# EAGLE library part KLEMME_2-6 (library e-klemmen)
Klemme 2 6
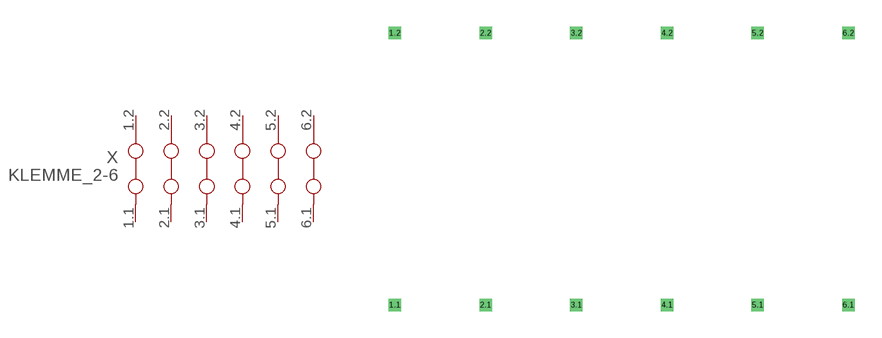
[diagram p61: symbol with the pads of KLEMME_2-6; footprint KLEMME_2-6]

Designator prefix X

## KLEMME_2-6  [KLEMME_2-6]
1.1  1.1  pas
1.2  1.2  pas
2.1  2.1  pas
2.2  2.2  pas
3.1  3.1  pas
3.2  3.2  pas
4.1  4.1  pas
4.2  4.2  pas
5.1  5.1  pas
5.2  5.2  pas
6.1  6.1  pas
6.2  6.2  pas

## Footprint KLEMME_2-6 (pad centres in mm)
Dummy
drill 0.2 pad 0.6 square: 1.1 0,-7.62; 1.2 0,7.62; 2.1 5.08,-7.62; 2.2 5.08,7.62; 3.1 10.16,-7.62; 3.2 10.16,7.62; 4.1 15.24,-7.62; 4.2 15.24,7.62; 5.1 20.32,-7.62; 5.2 20.32,7.62; 6.1 25.4,-7.62; 6.2 25.4,7.62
